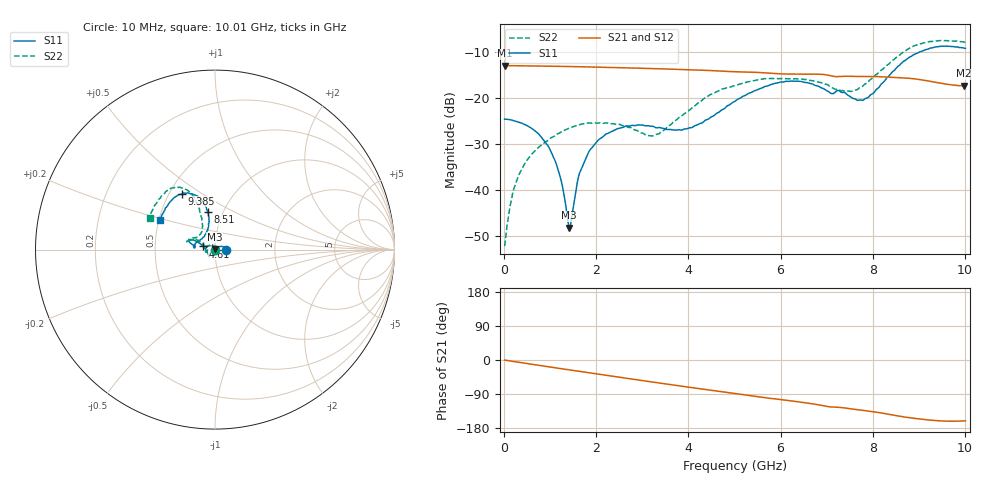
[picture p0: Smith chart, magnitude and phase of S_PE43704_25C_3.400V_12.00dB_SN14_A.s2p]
! Device ID: PE43704
! Dir: z:\PE43704\PE43704_Char_1_20130516\PE43704\AMB\3p400V\12p00dB
! Serial: 14
! Insertion: A
! Impedance: 50 ohm
! Temp: Amb
! VDD: 3.400V
! Attenuation Step: 12.00dB
! IDD: 1.139000e-01mA
#  Hz  S  RI  R  50
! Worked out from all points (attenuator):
!   401 points, 10 MHz to 10.01 GHz, reference 50 ohm
!   highest |S21| = -12.93 dB at 10 MHz (marker M1); lowest = -17.3 dB at 9.985 GHz (marker M2)
!   lowest |S11| = -48.2 dB at 1.41 GHz (marker M3), VSWR 1.01, Z = 49.8 + j0.322 ohm
!   |S11| at or under -10 dB: start of sweep to 9.009 GHz
!   |S22| runs from -52.3 to -7.5 dB; largest |S21 - S12| = 0.0016
!   S11 on the Smith chart (normalised r, x): 10 MHz: 1.12, +0.00; 4.61 GHz: 0.88, +0.03; 8.51 GHz: 0.85, +0.37; 9.385 GHz: 0.58, +0.42; 10.01 GHz: 0.51, +0.19
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1e7  0.0588 0.00016  0.2256 -0.000852  0.2258 -0.000775  0.0024 0.00041
1.6e8  0.0575 0.00478  0.2247 -0.0123  0.2247 -0.0122  0.00218 0.00752
3.1e8  0.0539 0.00962  0.2234 -0.0231  0.2233 -0.0231  -0.000279 0.0142
9.35e8  0.026 0.0168  0.2121 -0.0662  0.2122 -0.0661  -0.0229 0.0253
1.185e9  0.0109 0.0113  0.2054 -0.0827  0.2054 -0.0826  -0.0352 0.0214
1.41e9  -0.00213 0.00323  0.198 -0.0965  0.198 -0.0965  -0.0446 0.0148
1.46e9  -0.00456 0.0013  0.1963 -0.0995  0.1962 -0.0994  -0.0462 0.013
1.685e9  -0.0153 -0.00813  0.1878 -0.1128  0.1879 -0.1126  -0.0521 0.00454
1.885e9  -0.0226 -0.0166  0.1795 -0.1235  0.1796 -0.1234  -0.0531 -0.00274
2.26e9  -0.0288 -0.0298  0.1623 -0.1423  0.1623 -0.1422  -0.0521 -0.011
3.36e9  -0.0344 -0.0332  0.1022 -0.1815  0.1024 -0.1812  -0.0403 0.00568
4.01e9  -0.0464 -0.0087  0.0633 -0.1928  0.0635 -0.1928  -0.0671 0.0294
4.61e9  -0.0658 0.0175  0.027 -0.1958  0.0275 -0.1959  -0.1037 0.0545
5.01e9  -0.0853 0.0346  0.00491 -0.1935  0.00514 -0.1935  -0.1263 0.0533
5.96e9  -0.1361 0.0564  -0.044 -0.1786  -0.0435 -0.1789  -0.1546 0.0507
6.685e9  -0.1378 0.0366  -0.0783 -0.164  -0.0785 -0.164  -0.1457 0.0518
7.735e9  -0.0669 0.0677  -0.1152 -0.1274  -0.1149 -0.1275  -0.0723 0.1089
8.36e9  -0.0339 0.1729  -0.1358 -0.1005  -0.1352 -0.101  -0.086 0.222
8.51e9  -0.0379 0.208  -0.1397 -0.0913  -0.1391 -0.0921  -0.0991 0.258
9.385e9  -0.1823 0.3119  -0.1386 -0.0504  -0.1392 -0.0498  -0.2529 0.3347
9.985e9  -0.2999 0.1778  -0.1284 -0.0446  -0.1286 -0.0445  -0.3603 0.1862
1.001e10  -0.3051 0.1676  -0.1282 -0.0451  -0.1292 -0.0456  -0.3638 0.178
